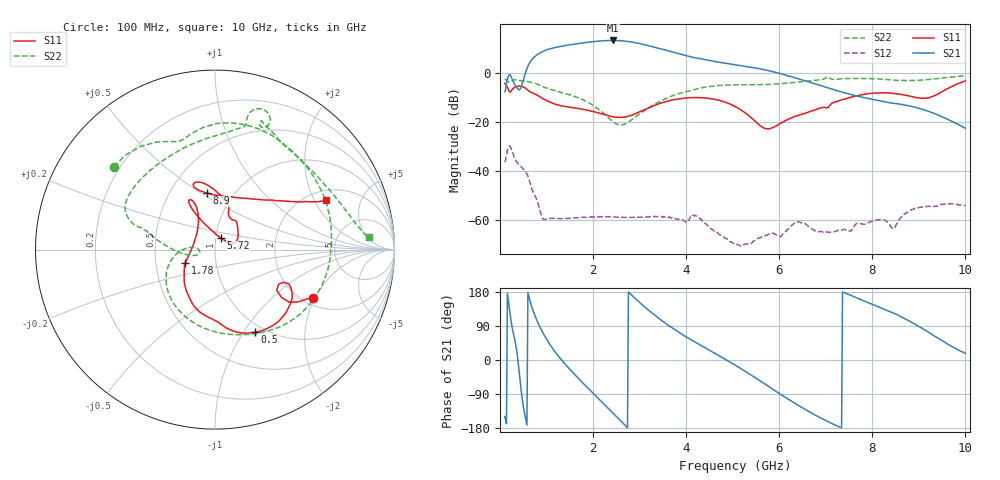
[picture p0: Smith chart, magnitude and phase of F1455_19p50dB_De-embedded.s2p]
! Integrated Device Technology
! Corporate Headquarters
! 6024 Silver Creek Valley Road
! San Jose, CA 95138  USA
! Phone:  1-408-284-8200
! Toll Free:  1-800-223-1366
! Webpage:  http://www.idt.com/
! Timing and RF Division
! 515 Groton Road, Suite 102
! Westford, MA 01886-6024
! Device:  F1455
! Description: 6-bit 0.5 dB Transmit Variable Gain Amplifier
! Frequency:  1400.0 -  2300.00 MHz
! Package:  6x6 mm Thin QFN Plastic Package: 28 pin
! State:  39
! Atten State:  19.5 dB
! Voltage:  +5.00 Volts
! Current:  217.612 mA
! Data:  The device was measured on a the F1455 evaluation board which has
!  individual transmission lines to the RF pins.  Data was collected
!  using a calibrated network analyzer.  The evaluation board was
!  de-embedded using a TRL calibration technique.
!  The reference plane is the edge of the package pin.
!  Pin  1 = CSb
!  Pin  2 = DATA
!  Pin  3 = CLK
!  Pin  4 = RSET
!  Pin  5 = GND
!  Pin  6 = RFIN  = Port 1
!  Pin  7 = GND
!  Pin  8 = NC
!  Pin  9 = NC
!  Pin 10 = NC
!  Pin 11 = NC
!  Pin 12 = NC
!  Pin 13 = NC
!  Pin 14 = /STBY
!  Pin 15 = GND
!  Pin 16 = RFOUT  = Port 2
!  Pin 17 = GND
!  Pin 18 = NC
!  Pin 19 = NC
!  Pin 20 = NC
!  Pin 21 = GND
!  Pin 22 = NC
!  Pin 23 = GND
!  Pin 24 = NC
!  Pin 25 = NC
!  Pin 26 = NC
!  Pin 27 = GND
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# GHz S dB R 50
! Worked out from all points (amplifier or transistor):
!   496 points, 100 MHz to 10 GHz, reference 50 ohm
!   highest |S21| = 13.1 dB at 2.42 GHz (marker M1)
!   |S21| within 3 dB of that: 1.16 GHz to 3.376 GHz (2.216 GHz wide, 97.7 % of centre)
!   unconditionally stable (mu >= 1): start of sweep to end of sweep
!   at 1.74 GHz: K = 96.82, MAG = 12.5 dB, |S12| = -58.8 dB
!   at 5.06 GHz: K = 720.66, MAG = 5.1 dB, |S12| = -70.1 dB
!   at 10 GHz: K = 471.27, MAG = -14.0 dB, |S12| = -54.1 dB
!   S11 on the Smith chart (normalised r, x): 100 MHz: 2.26, -1.92; 500 MHz: 0.91, -1.13; 1.78 GHz: 0.71, -0.11; 5.72 GHz: 1.06, +0.14; 8.9 GHz: 0.76, +0.53; 10 GHz: 2.47, +2.50
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0.1  -4.33 -26.2  -7.68 -148.9  -36.32 46.8  -2.76 140.7
0.26  -6.90 -24.8  -2.50 87.1  -31.88 -76.6  -3.31 95.7
0.38  -5.53 -41.9  -6.51 5.7  -36.76 -116.7  -3.06 57.8
0.5  -5.82 -64.1  -3.11 -120.5  -39.15 -155.1  -3.39 27.1
0.68  -8.11 -90.6  5.20 142.0  -46.89 139.6  -3.97 -14.4
0.82  -9.36 -108.9  7.58 97.0  -53.31 112.5  -4.82 -45.5
0.96  -10.94 -123.4  8.97 63.8  -59.82 125.9  -5.99 -70.8
1.34  -13.53 -144.6  10.81 -2.3  -59.35 97.4  -8.12 -121.1
1.76  -14.81 -155.7  12.06 -58.0  -58.78 64.5  -10.82 -157.7
1.78  -14.90 -156.3  12.11 -60.4  -58.80 63.3  -11.00 -159.1
2.1  -16.26 -165.9  12.81 -99.6  -58.61 46.4  -14.61 -179.0
2.42  -17.86 175.3  13.10 -139.1  -58.67 32.2  -19.78 175.7
2.8  -17.51 140.2  12.54 174.6  -58.91 20.6  -19.58 -163.7
3.1  -15.08 121.6  11.41 140.9  -58.74 13.4  -15.48 -171.4
3.4  -12.75 114.7  9.97 111.0  -58.46 3.0  -12.05 177.9
4.08  -10.18 116.1  6.54 55.3  -59.17 -8.9  -7.38 163.5
5.06  -13.80 117.1  3.21 -14.0  -70.13 -31.0  -4.93 148.5
5.72  -22.79 62.2  1.03 -65.5  -66.18 -1.6  -4.82 121.3
6.7  -15.60 39.4  -4.14 -140.4  -63.52 -132.5  -3.22 78.6
8.36  -8.25 107.8  -12.19 128.5  -61.57 101.6  -2.83 62.6
8.9  -9.98 98.2  -13.99 95.6  -55.37 117.0  -3.18 41.1
10  -3.37 23.8  -22.56 17.5  -54.12 38.8  -1.29 4.6
